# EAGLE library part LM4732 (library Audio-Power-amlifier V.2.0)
The LM4732 is a stereo audio amplifier capable of typically delivering 50W per channel of continuous average output power into a 4Ω or 8Ω load with less than 10% THD+N from 20Hz - 20kHz
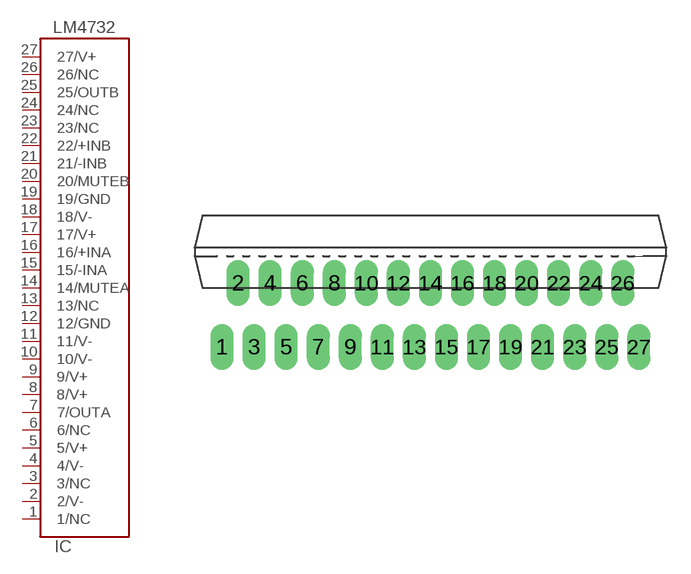
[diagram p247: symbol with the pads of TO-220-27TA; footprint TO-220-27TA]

Designator prefix IC

## LM4732  [TO-220-27TA]
1  1/NC  nc
2  2/V-  pwr
3  3/NC  nc
4  4/V-  pwr
5  5/V+  pwr
6  6/NC  nc
7  7/OUTA  out
8  8/V+  pwr
9  9/V+  pwr
10  10/V-  pwr
11  11/V-  pwr
12  12/GND  pwr
13  13/NC  nc
14  14/MUTEA  in
15  15/-INA  in
16  16/+INA  in
17  17/V+  pwr
18  18/V-  pwr
19  19/GND  pwr
20  20/MUTEB  in
21  21/-INB  in
22  22/+INB  in
23  23/NC  nc
24  24/NC  nc
25  25/OUTB  out
26  26/NC  nc
27  27/V+  pwr

## Footprint TO-220-27TA (pad centres in mm)
TO-220_MKT-TA27A , MOLDED (inch. 1,150x0,618x0,177 - body_0,040 pitch )
drill 0.5 pad 1.422 long: 1 -13.007,-3.988; 2 -12.009,0; 3 -11.008,-3.988; 4 -10.008,0; 5 -9.007,-3.988; 6 -8.006,0; 7 -7.005,-3.988; 8 -6.002,0; 9 -5.004,-3.988; 10 -4.003,0; 11 -3.002,-3.988; 12 -1.999,0; 13 -1.001,-3.99; 14 0,0; 15 1.001,-3.988; 16 2.002,0; 17 3.002,-3.988; 18 4.003,0; 19 5.004,-3.988; 20 6.007,0; 21 7.005,-3.988; 22 8.006,0; 23 9.009,-3.988; 24 10.008,0; 25 11.008,-3.988; 26 12.009,0; 27 13.01,-3.988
